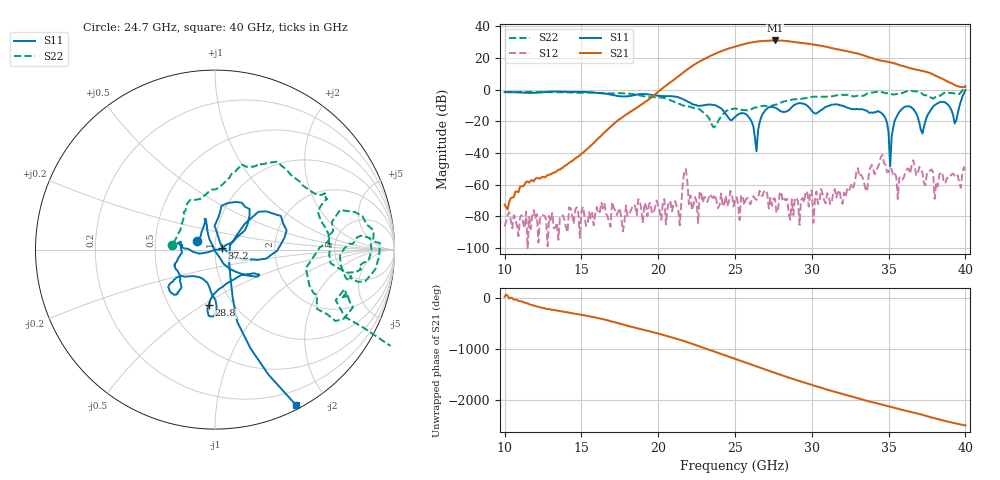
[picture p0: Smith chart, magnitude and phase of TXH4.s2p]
!Keysight Technologies,M9808A,MY58100618,A.14.70.03
!Date: Monday, February 27, 2023 13:18:32
!Correction: S11(C  2-Port  )
!S21(C  2-Port  )
!S12(C  2-Port  )
!S22(C  2-Port  )
!S2P File: Measurements: S11, S21, S12, S22:
# Hz S  RI  R 50
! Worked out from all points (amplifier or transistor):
!   301 points, 10 GHz to 40 GHz, reference 50 ohm
!   highest |S21| = 31.1 dB at 27.6 GHz (marker M1)
!   |S21| within 3 dB of that: 25.33 GHz to 30.43 GHz (5.098 GHz wide, 18.3 % of centre)
!   unconditionally stable (mu >= 1): start of sweep to 39.84 GHz
!   at 15 GHz: K = 38546.08, MAG = -30.7 dB, |S12| = -76.9 dB
!   at 25 GHz: K = 64.24, MAG = 27.6 dB, |S12| = -70.1 dB
!   at 40 GHz: K = -7.58, MSG = 26.7 dB, |S12| = -51.7 dB
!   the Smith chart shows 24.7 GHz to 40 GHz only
!   S11 on the Smith chart (normalised r, x): 24.7 GHz: 0.82, +0.08; 28.8 GHz: 0.77, -0.53; 37.2 GHz: 1.08, +0.02; 40 GHz: 0.04, -1.65
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1e10  0.7597 0.3343  0.000196 0.000125  4.12e-05 2.34e-05  -0.0141 0.8531
1.5e10  0.6119 -0.5844  0.00742 0.0057  -1.07e-05 0.000143  0.7411 0.2965
2e10  -0.1628 -0.6201  0.7502 0.4202  -0.000176 0.000114  0.272 -0.5052
2.25e10  -0.3054 -0.0975  -6.244 2.734  0.000225 -0.000192  -0.0282 -0.2551
2.34e10  -0.3378 -0.00786  5.49 10.22  4.94e-05 0.000501  -0.0108 -0.1038
2.41e10  -0.2522 -0.0398  15.97 -3.486  0.000526 7.14e-06  -0.1365 0.0189
2.47e10  -0.0983 0.0485  4.872 -20.09  -0.000355 -0.000524  -0.2418 0.0275
2.5e10  -0.0668 0.1191  -7.124 -21.73  -0.000289 0.000117  -0.2536 0.0307
2.58e10  -0.0478 0.147  -28.38 6.593  -0.000373 7.3e-05  -0.1925 0.1088
2.65e10  0.0259 -0.0442  -0.8053 33.32  -0.000246 -0.000271  -0.1597 0.237
2.71e10  0.2073 -0.1479  30.78 16.13  0.00033 -0.000393  -0.106 0.2782
2.76e10  0.2326 -0.1377  32.37 -15.2  -7.8e-05 0.000355  -0.02 0.3334
2.82e10  0.1016 -0.1685  1.445 -34.82  0.000311 -0.000184  0.0884 0.4169
2.88e10  -0.0346 -0.3104  -27.32 -17.2  -0.000102 -3.69e-05  0.1425 0.4728
2.93e10  -0.00505 -0.3718  -28.84 7.691  0.000305 0.000104  0.2152 0.4622
3e10  -0.0301 -0.2117  -3.842 26.78  -0.000245 -0.000615  0.3304 0.4875
3.08e10  -0.2111 -0.1546  21.4 9.274  0.000308 -9.52e-05  0.4221 0.4172
3.19e10  -0.2087 -0.2379  5.345 -16.96  -0.000292 -0.000173  0.6082 0.3105
3.3e10  -0.2242 -0.0962  -13.3 -3.274  0.00326 -0.00057  0.6338 0.0814
3.5e10  -0.0405 -0.0152  6.014 4.557  -0.000352 0.00246  0.7652 0.0305
3.72e10  0.04 0.0102  -2.494 -2.992  0.00245 -0.000175  0.6967 0.2203
4e10  0.4512 -0.8663  1.147 0.4143  -0.000996 -0.00242  1.203 -0.6486
